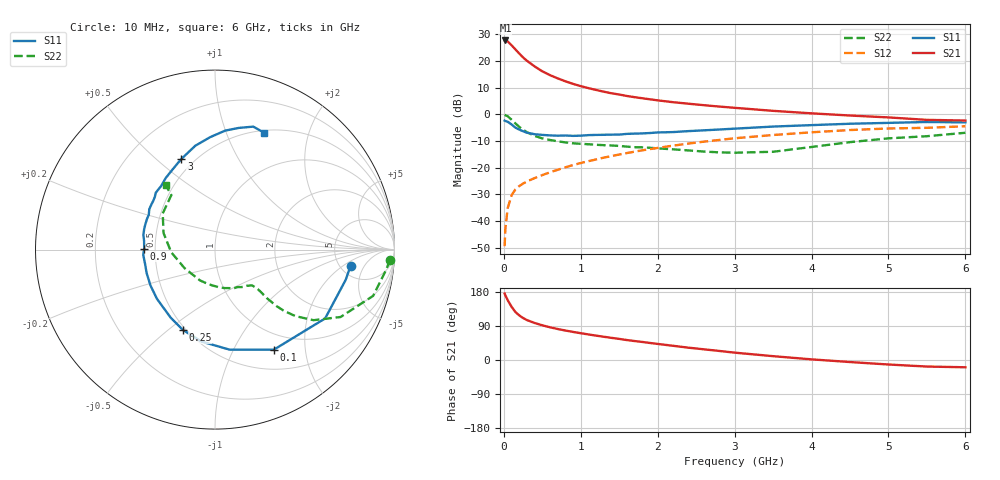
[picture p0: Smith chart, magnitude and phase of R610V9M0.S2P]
! SIEMENS Small Signal Semiconductors
! BFR193
! Si NPN RF Bipolar Junction Transistor in SOT23
! VCE = 10 V  IC = 9 mA
! Common Emitter S-Parameters:  May  1996
# GHz  S  MA  R  50
!  f  S11  S21  S12  S22
! GHz  MAG  ANG  MAG  ANG  MAG  ANG  MAG  ANG
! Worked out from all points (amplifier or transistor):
!   36 points, 10 MHz to 6 GHz, reference 50 ohm
!   highest |S21| = 27.6 dB at 20 MHz (marker M1)
!   |S21| within 3 dB of that: start of sweep to 139.2 MHz
!   unconditionally stable (mu >= 1): 800.6 MHz to 2 GHz
!   at 250 MHz: K = 0.59, MSG = 23.6 dB, |S12| = -25.9 dB
!   at 1.4 GHz: K = 1.04, MAG = 10.5 dB, |S12| = -15.7 dB
!   at 6 GHz: K = 0.94, MSG = 1.1 dB, |S12| = -4.5 dB
!   S11 on the Smith chart (normalised r, x): 10 MHz: 6.24, -2.63; 100 MHz: 0.76, -1.46; 250 MHz: 0.48, -0.56; 900 MHz: 0.43, +0.01; 3 GHz: 0.43, +0.61; 6 GHz: 0.53, +1.37
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0.01  0.7612 -6.7  24.09 175.3  0.0034 80.9  0.9763 -3.3
0.02  0.7475 -13.0  24.1 170.6  0.0072 80.1  0.9609 -6.6
0.05  0.7237 -32.0  23.07 157.9  0.0175 73.9  0.9181 -16.3
0.1  0.6468 -59.6  19.64 140.6  0.0304 65.6  0.7944 -28.2
0.15  0.5634 -81.7  16.41 126.8  0.0393 57.8  0.6757 -35.6
0.2  0.5178 -98.4  13.73 117.7  0.0453 55.5  0.5815 -39.6
0.25  0.4817 -111.9  11.59 110.8  0.0505 54.3  0.5141 -41.6
0.3  0.4521 -123.2  10.05 105.4  0.0552 54.5  0.4637 -42.6
0.4  0.424 -139.8  7.875 97.7  0.064 55.7  0.3942 -43.1
0.5  0.4112 -151.1  6.374 91.5  0.0727 57.2  0.3536 -42.8
0.6  0.4027 -161.0  5.402 86.3  0.0821 58.4  0.3307 -42.7
0.7  0.3977 -168.7  4.703 81.8  0.0915 59.8  0.3126 -43.0
0.9  0.3945 179.2  3.707 74.1  0.1122 61.3  0.2863 -44.1
1.1  0.4075 168.3  3.086 67.4  0.1326 61.6  0.2749 -47.1
1.3  0.413 159.8  2.646 61.3  0.1547 61.2  0.2641 -50.3
1.6  0.4299 148.4  2.201 52.6  0.1881 59.9  0.2482 -57.3
2.2  0.4644 130.2  1.684 37.5  0.2591 54.9  0.2208 -76.1
3  0.5385 110.4  1.322 19.4  0.3556 44.9  0.1909 -116.2
3.5  0.5892 100.7  1.16 10.1  0.4094 37.7  0.1988 -148.8
4.5  0.6654 85.1  0.948 -5.4  0.5074 23.0  0.3011 162.2
5.5  0.7176 72.7  0.786 -17.3  0.5584 7.4  0.389 128.7
6  0.7063 67.1  0.764 -19.2  0.5977 2.9  0.4508 127.4
